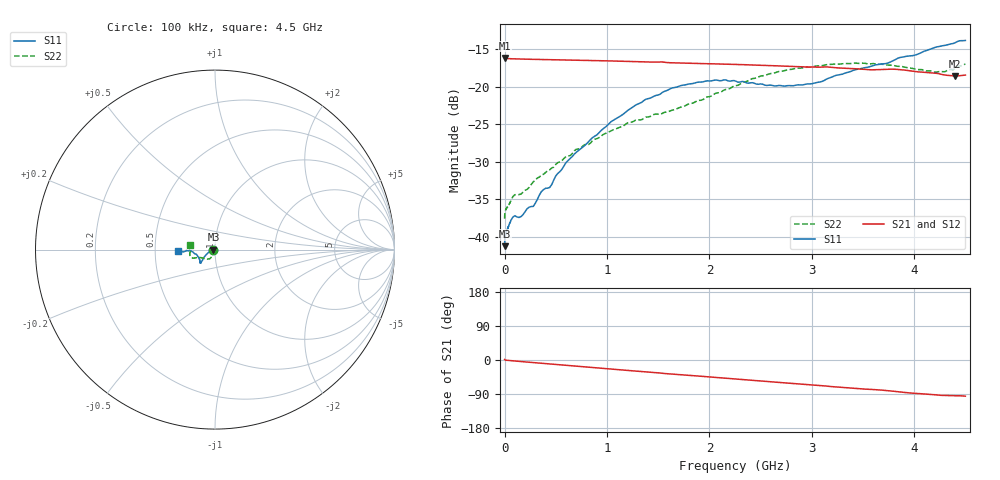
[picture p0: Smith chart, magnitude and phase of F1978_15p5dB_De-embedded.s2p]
! Integrated Device Technology
! Corporate Headquarters
! 6024 Silver Creek Valley Road
! San Jose, CA 95138  USA
! Phone:  1-408-284-8200
! Toll Free:  1-800-223-1366
! Webpage:  http://www.idt.com/
! Timing and RF Division
! 515 Groton Road, Suite 102
! Westford, MA 01886-6024
! Device:  F1978
! Description: 6-bit, 75 ohm, 0.5 dB Digital Step Attenuator
! Frequency:  5.0 MHz -  3.00 GHz
! Package:  4x4 mm QFN Plastic Package: 20 pin
! Ports:  2 RF, 11 DC
!  Pin  1  = D5 (16 dB)
!  Pin  2  = RF1  =  Port 1
!  Pin  3  = Serial Data In (DATA)
!  Pin  4  = Serial Clock (CLK)
!  Pin  5  = Serial Latch Enable (LE)
!  Pin  6  = VDD
!  Pin  7  = NC
!  Pin  8  = NC
!  Pin  9  = NC
!  Pin 10  = GND
!  Pin 11  = GND
!  Pin 12  = NC
!  Pin 13  = VMODE
!  Pin 14  = RF2  =  Port 2
!  Pin 15  = D4 (8 dB)
!  Pin 16  = D3 (4 dB)
!  Pin 17  = D2 (2 dB)
!  Pin 18  = NC
!  Pin 19  = D1 (1 dB)
!  Pin 20  = D0 (0.5 dB)
! State:  31
! Atten State:  15.5 dB
! Voltage:  +3.30 Volts
! Current:  0.563 mA
! Data:  The device was measured on a F1975 evaluation board which has
!  individual transmission lines to the RF pins.  Data was collected
!  using a calibrated network analyzer.  The evaluation board was
!  de-embedded using Automatic Fixture Removal (AFR).
!  The reference plane is the edge of the package pin.
! Misc:
!  Action Tracker AT0416
! Date Measured:  2018-02-08
! Date:  2018-03-26  MJV
! Note:
!  Integrated Device Technology supplies this data as a sample of measured
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# GHz S dB R 75
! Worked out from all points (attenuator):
!   291 points, 100 kHz to 4.5 GHz, reference 75 ohm
!   highest |S21| = -16.13 dB at 100 kHz (marker M1); lowest = -18.5 dB at 4.4 GHz (marker M2)
!   lowest |S11| = -41.3 dB at 100 kHz (marker M3), VSWR 1.02, Z = 73.7 - j0.00784 ohm
!   |S11| at or under -10 dB: start of sweep to end of sweep
!   |S22| runs from -37.6 to -16.8 dB; largest |S21 - S12| = 0.00015
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0.0001  -41.28 -179.6  -16.13 1.2  -16.13 1.2  -37.61 -178.5
0.0005  -40.68 -177.8  -16.15 1.1  -16.15 1.1  -37.33 -177.9
0.003  -40.14 -175.9  -16.18 0.7  -16.17 0.7  -36.83 -176.4
0.014  -39.46 -174.8  -16.21 -0.6  -16.21 -0.6  -36.37 -173.3
0.08  -37.42 -168.5  -16.25 -2.2  -16.25 -2.2  -34.68 -161.8
0.16  -37.33 -166.0  -16.29 -4.1  -16.29 -4.1  -34.32 -146.9
0.28  -35.97 -165.5  -16.32 -6.8  -16.32 -6.8  -32.70 -136.2
0.36  -33.98 -165.3  -16.35 -8.6  -16.34 -8.6  -31.77 -128.2
0.44  -33.44 -163.1  -16.36 -10.4  -16.36 -10.4  -31.09 -122.7
0.6  -30.11 -161.3  -16.41 -14.0  -16.41 -14.0  -29.32 -119.3
0.76  -28.09 -155.2  -16.45 -17.6  -16.45 -17.6  -27.95 -117.6
1.04  -24.65 -149.6  -16.54 -23.9  -16.53 -23.9  -25.86 -117.2
1.38  -21.65 -143.3  -16.67 -31.4  -16.67 -31.4  -24.04 -123.7
1.52  -20.97 -140.1  -16.68 -34.4  -16.67 -34.4  -23.65 -127.4
1.88  -19.39 -137.1  -16.87 -42.1  -16.87 -42.1  -21.87 -142.6
2.26  -19.25 -138.7  -17.00 -50.2  -17.00 -50.2  -19.83 -154.1
2.64  -19.89 -149.1  -17.18 -58.3  -17.18 -58.3  -18.13 -157.8
3.02  -19.51 -164.3  -17.36 -66.0  -17.35 -66.0  -17.28 -160.9
3.76  -16.72 -177.2  -17.63 -81.3  -17.63 -81.3  -17.11 -174.2
4.2  -14.74 -176.0  -18.17 -91.7  -18.17 -91.7  -18.03 174.2
4.4  -14.10 -175.0  -18.54 -94.3  -18.54 -94.3  -17.58 171.2
4.5  -13.80 -177.0  -18.43 -95.5  -18.42 -95.5  -16.92 169.8
